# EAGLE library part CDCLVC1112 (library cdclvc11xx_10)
CDCLVC1112 3.3V and 2.5V LVCMOS High-Performance Clock Buffer - 1:12 Fan-out Source: http://www.ti.com/lit/ds/symlink/cdclvc1112.pdf
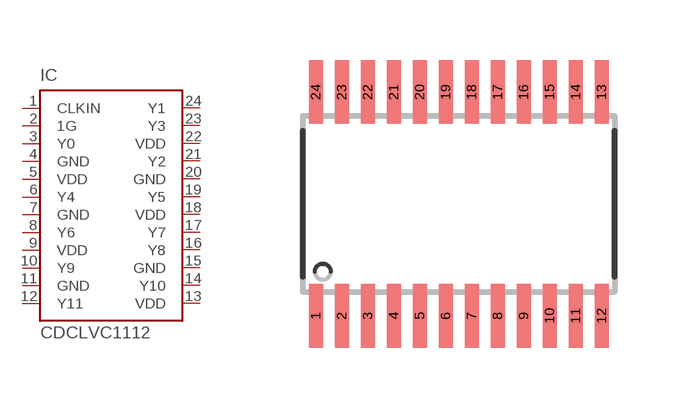
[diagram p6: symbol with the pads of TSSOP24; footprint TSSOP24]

Designator prefix IC

## CDCLVC1112PW (MF: Texas Instruments; MPN: CDCLVC1112; OC_FARNELL: 1829667; OC_NEWARK: 77R3941)  [TSSOP24]
1  CLKIN  in
2  1G  in
3  Y0  out
4  GND  pwr
5  VDD  pwr
6  Y4  out
7  GND  pwr
8  Y6  out
9  VDD  pwr
10  Y9  out
11  GND  pwr
12  Y11  out
13  VDD  pwr
14  Y10  out
15  GND  pwr
16  Y8  out
17  Y7  out
18  VDD  pwr
19  Y5  out
20  GND  pwr
21  Y2  out
22  VDD  pwr
23  Y3  out
24  Y1  out

## Footprint TSSOP24 (pad centres in mm)
TSSOP-24 Plastic Thin Srink Small Outline (PW) Source: http://www.ti.com/lit/ds/symlink/cdclvc1112.pdf
smd 0.35 x 1.6: 1 -3.575,-2.8; 2 -2.925,-2.8; 3 -2.275,-2.8; 4 -1.625,-2.8; 5 -0.975,-2.8; 6 -0.325,-2.8; 7 0.325,-2.8; 8 0.975,-2.8; 9 1.625,-2.8; 10 2.275,-2.8; 11 2.925,-2.8; 12 3.575,-2.8; 13 3.575,2.8; 14 2.925,2.8; 15 2.275,2.8; 16 1.625,2.8; 17 0.975,2.8; 18 0.325,2.8; 19 -0.325,2.8; 20 -0.975,2.8; 21 -1.625,2.8; 22 -2.275,2.8; 23 -2.925,2.8; 24 -3.575,2.8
